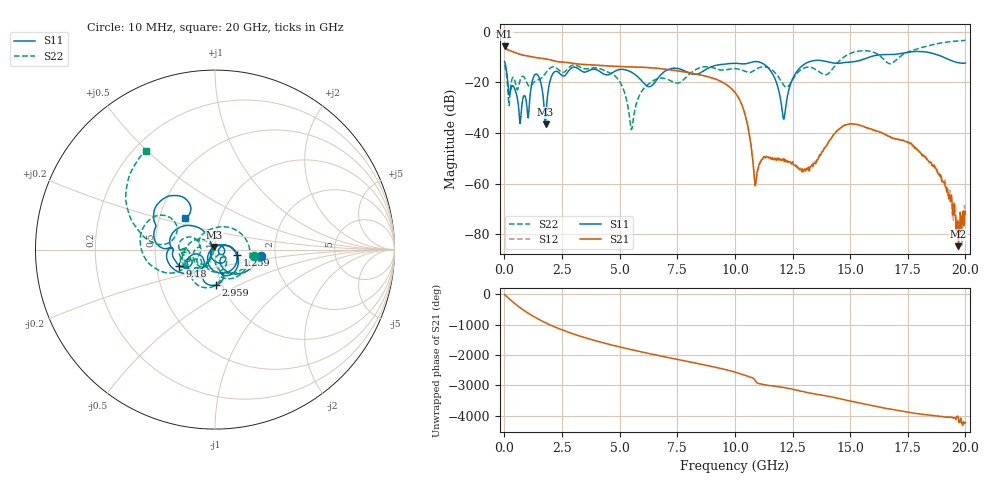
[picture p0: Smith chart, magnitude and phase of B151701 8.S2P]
!  2-Port S-parameters saved by WinCal
! VAR MeasName=S-Parameters (CALIBRATED_DATA) read from VNA (N5244A)
! VAR MeasDate=2015-12-24 19:09:00
! VAR NAME=B151701 8
! VAR FILENAME=B151701 8.S2P
! VAR DATE=2015-12-24 19:09:00
! VAR PHYS_PORTS=1,3
# Hz S DB R 50
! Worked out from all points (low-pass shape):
!   801 points, 10 MHz to 20 GHz, reference 50 ohm
!   highest |S21| = -5.83 dB at 10 MHz (marker M1); lowest = -84.6 dB at 19.7 GHz (marker M2)
!   |S21| within 3 dB of the highest: start of sweep to 653.7 MHz
!   lowest |S11| = -36.5 dB at 1.784 GHz (marker M3), VSWR 1.03, Z = 49.6 + j1.42 ohm
!   |S11| at or under -10 dB: start of sweep to 15.86 GHz; 19.04 GHz to end of sweep
!   |S22| runs from -38.7 to -3.5 dB; largest |S21 - S12| = 0.0011
!   S11 on the Smith chart (normalised r, x): 10 MHz: 1.68, -0.12; 1.259 GHz: 1.28, -0.08; 2.959 GHz: 0.93, -0.38; 9.18 GHz: 0.66, -0.12; 20 GHz: 0.68, +0.25
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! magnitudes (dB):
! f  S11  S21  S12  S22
! 10 MHz  -11.8  -5.8  -5.8  -13.1
! 209.9 MHz  -25.0  -7.4  -7.4  -29.2
! 684.7 MHz  -36.3  -8.9  -8.9  -19.1
! 1.259 GHz  -18.0  -10.1  -10.1  -20.1
! 1.784 GHz  -36.5  -10.7  -10.7  -16.4
! 2.109 GHz  -16.5  -11.4  -11.4  -13.9
! 2.959 GHz  -14.1  -12.4  -12.4  -13.2
! 3.358 GHz  -15.6  -12.9  -12.9  -14.3
! 4.883 GHz  -15.2  -13.7  -13.7  -18.3
! 5.507 GHz  -15.9  -13.9  -13.9  -38.7
! 6.682 GHz  -18.1  -14.5  -14.5  -18.4
! 9.18 GHz  -13.3  -18.8  -18.8  -14.6
! 10.01 GHz  -12.5  -24.0  -24.0  -14.6
! 10.48 GHz  -12.6  -34.2  -34.0  -15.8
! 10.9 GHz  -11.8  -59.9  -60.1  -14.9
! 12.13 GHz  -34.5  -50.1  -51.2  -21.2
! 13.35 GHz  -11.5  -52.5  -52.3  -14.2
! 14.8 GHz  -12.1  -36.8  -36.7  -9.5
! 16.68 GHz  -9.0  -41.3  -41.3  -12.6
! 18.6 GHz  -8.6  -52.9  -52.8  -5.1
! 19.7 GHz  -12.3  -84.6  -74.7  -3.6
! 20 GHz  -12.4  -72.0  -71.1  -3.5
